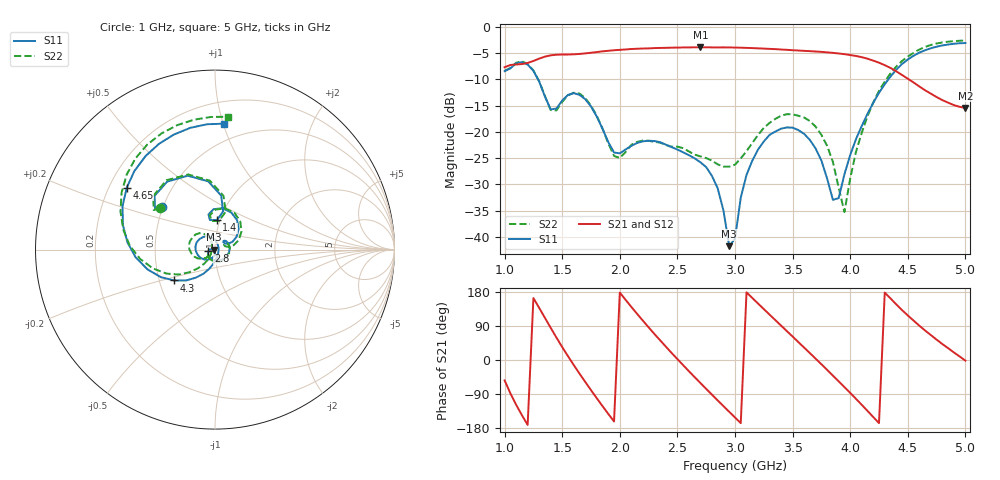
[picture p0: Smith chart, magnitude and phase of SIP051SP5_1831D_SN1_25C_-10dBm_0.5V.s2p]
# GHz  S  dB  R  50
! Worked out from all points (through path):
!   81 points, 1 GHz to 5 GHz, reference 50 ohm
!   highest |S21| = -3.87 dB at 2.7 GHz (marker M1); lowest = -15.4 dB at 5 GHz (marker M2)
!   lowest |S11| = -41.8 dB at 2.95 GHz (marker M3), VSWR 1.02, Z = 49.2 - j0.042 ohm
!   |S11| at or under -10 dB: 1.291 GHz to 4.331 GHz (3.04 GHz wide, 108 % of centre)
!   |S22| runs from -35.3 to -2.6 dB; largest |S21 - S12| = 0.0028
!   S11 on the Smith chart (normalised r, x): 1 GHz: 0.49, +0.27; 1.4 GHz: 0.97, +0.33; 2.8 GHz: 0.93, -0.02; 4.3 GHz: 0.60, -0.22; 4.65 GHz: 0.27, +0.29; 5 GHz: 0.36, +1.01
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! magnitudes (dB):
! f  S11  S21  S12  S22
! 1 GHz  -8.4  -7.7  -7.7  -8.3
! 1.2 GHz  -7.2  -6.8  -6.8  -7.0
! 1.4 GHz  -15.7  -5.4  -5.4  -15.8
! 1.7 GHz  -13.8  -5.0  -5.0  -13.5
! 1.95 GHz  -23.9  -4.4  -4.4  -24.6
! 2.35 GHz  -21.9  -4.0  -4.0  -22.0
! 2.7 GHz  -25.8  -3.9  -3.9  -24.7
! 2.8 GHz  -28.4  -3.9  -3.9  -25.5
! 2.9 GHz  -35.0  -3.9  -3.9  -26.6
! 2.95 GHz  -41.8  -3.9  -3.9  -26.6
! 3 GHz  -40.3  -3.9  -3.9  -26.2
! 3.1 GHz  -28.2  -4.0  -4.0  -23.7
! 3.3 GHz  -20.6  -4.2  -4.2  -18.3
! 3.5 GHz  -19.2  -4.4  -4.4  -16.6
! 3.7 GHz  -23.2  -4.7  -4.7  -19.0
! 3.85 GHz  -32.9  -4.9  -4.9  -25.7
! 3.95 GHz  -28.1  -5.2  -5.2  -35.3
! 4.1 GHz  -18.9  -5.7  -5.7  -20.2
! 4.3 GHz  -10.9  -7.3  -7.3  -10.4
! 4.35 GHz  -9.4  -7.8  -7.8  -8.8
! 4.65 GHz  -4.4  -12.1  -12.1  -3.8
! 5 GHz  -3.1  -15.4  -15.4  -2.6
